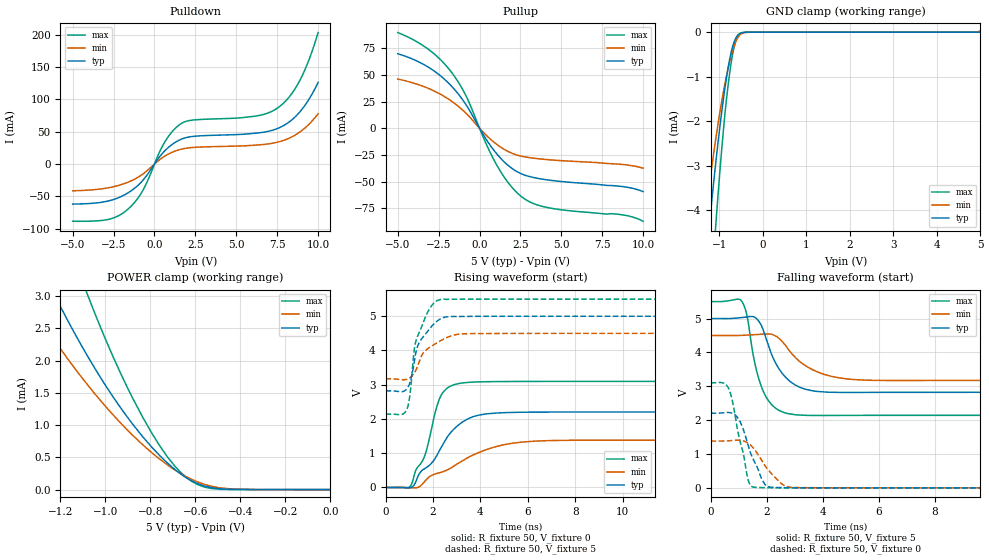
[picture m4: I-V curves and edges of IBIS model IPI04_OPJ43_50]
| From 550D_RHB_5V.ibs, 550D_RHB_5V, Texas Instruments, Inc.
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[Model]   IPI04_OPJ43_50
Model_type  I/O
Vinl = 0
Vinh = 5
Enable   Active-Low
Vref =   2.5
Rref =   50
Cref =   15p
Vmeas =   2.5
| variable   typ   min   max
C_comp   0.72pF   0.63pF   0.83pF
| C_pullup   1.77pF   0.56pF   2.42pF
| C_pulldown   1.53pF   0.86pF   2.26pF
| C_tri-state   0.72pF   0.63pF   0.83pF
[Temperature Range]   40   125   -40
| Ambient temperature   25   110   -40
[Voltage range]   5   4.5   5.5
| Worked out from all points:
|   slope of the pulldown table from 0 to 0.75 V, typ, clamps not added: 32.2 ohm
|   slope of the pullup table from 0 to 0.75 V, typ, clamps not added: 41.5 ohm
|   GND clamp passes 1 mA (typ) near -0.83 V on its own axis
|   POWER clamp passes 1 mA (typ) near -0.88 V on its own axis
|   rising waveform, R_fixture 50, V_fixture 0: 20-80 % time 1.51ns typ, 2.47ns min, 828ps max; typ from 0 V to 2.2 V
|   falling waveform, R_fixture 50, V_fixture 5: 20-80 % time 767ps typ, 1.13ns min, 547ps max; typ from 5 V to 2.82 V
|   rising waveform, R_fixture 50, V_fixture 5: 20-80 % time 679ps typ, 908ps min, 550ps max; typ from 2.82 V to 5 V
|   falling waveform, R_fixture 50, V_fixture 0: 20-80 % time 590ps typ, 746ps min, 451ps max; typ from 2.2 V to 0 V
[GND Clamp]
| IPI04_OPJ43_50
|   Voltage   I(typ)   I(min)   I(max)
-5V       -60.97mA   -47mA      -82.47mA
-1.345V   -5.553mA   -4.338mA   -8.207mA
-1.245V   -4.505mA   -3.561mA   -6.669mA
-1.205V   -4.104mA   -3.264mA   -6.077mA
-1.09V    -3.015mA   -2.458mA   -4.458mA
-1.055V   -2.704mA   -2.228mA   -3.994mA
-890mV    -1.395mA   -1.259mA   -2.04mA
-765mV    -627.7uA   -676.6uA   -948.2uA
-705mV    -363.7uA   -454uA     -561.7uA
-630mV    -151.5uA   -236uA     -226.2uA
-500mV    -18.16uA   -39.39uA   -19.17uA
5V        193pA      32.25uA    129.3pA
[POWER Clamp]
| IPI04_OPJ43_50
|   Voltage   I(typ)   I(min)   I(max)
-5V       60.35mA    45.31mA    80.38mA
-1.38V    4.15mA     3.131mA    6.161mA
-1.35V    3.917mA    2.964mA    5.812mA
-1.23V    3.04mA     2.33mA     4.491mA
-1.08V    2.071mA    1.626mA    3.023mA
-935mV    1.28mA     1.041mA    1.82mA
-835mV    822.7uA    697.6uA    1.127mA
-725mV    413.9uA    384.1uA    510.5uA
-635mV    172.1uA    190uA      174.4uA
-560mV    55.87uA    81.45uA    39.27uA
-490mV    12.95uA    27.01uA    5.254uA
-84.4fV   193pA      729pA      150.2pA
[Pulldown]
| IPI04_OPJ43_50
|   Voltage   I(typ)   I(min)   I(max)
-5V       -61.89mA   -41.4mA    -88.4mA
-2.815V   -57.01mA   -36.69mA   -85.54mA
-1.595V   -44.17mA   -27.83mA   -69.1mA
-685mV    -24.41mA   -14.96mA   -39.62mA
685mV     21.77mA    13.02mA    36.26mA
1.68V     38.72mA    23.14mA    63.14mA
6.295V    47.91mA    29.41mA    74.47mA
7.65V     56.24mA    34.57mA    88.8mA
8.3V      66.21mA    40.68mA    105.5mA
8.9V      80.88mA    49.68mA    129.8mA
9.46V     100.5mA    61.8mA     161.9mA
10V       126mA      77.5mA     203mA
[Pullup]
| IPI04_OPJ43_50
|   Voltage   I(typ)   I(min)   I(max)
-5V       69.87mA    46.14mA    89.69mA
-3.13V    57.25mA    37.38mA    74.02mA
-1.7V     39.22mA    25.25mA    52.2mA
-795mV    21.32mA    13.58mA    29.33mA
360mV     -9.264mA   -5.829mA   -13.14mA
1.06V     -24.13mA   -15.16mA   -34.71mA
1.825V    -35.8mA    -22.32mA   -52.46mA
2.6V      -42.96mA   -26.31mA   -64.49mA
3.275V    -46.05mA   -27.96mA   -70.42mA
4.195V    -48.49mA   -29.43mA   -74.43mA
8.695V    -54.54mA   -33.87mA   -81.04mA
10V       -59.36mA   -37.37mA   -87.19mA
[Ramp]
| IPI04_OPJ43_50
| variable   typ   min   max
dV/dt_r   1.33/1.52E-09   0.84/2.50E-09   1.86/8.41E-10
dV/dt_f   1.34/7.91E-10   0.82/1.16E-09   2.06/5.58E-10
R_load = 50
[Rising Waveform]
| IPI04_OPJ43_50
R_fixture =   50
C_fixture =   0
L_fixture =   0
V_fixture =   0
V_fixture_min = 0
V_fixture_max = 0
|   Time   V(typ)   V(min)   V(max)
0s        -402.9nV   -5.07uV    340.7nV
1.045ns   -5.03mV    -6.704mV   34.55mV
1.285ns   183.1mV    -8.556mV   515.3mV
1.68ns    565.1mV    201.2mV    981.7mV
2.075ns   832.2mV    390.3mV    2.144V
2.31ns    1.126V     437.9mV    2.644V
3.11ns    1.845V     724.3mV    3.038V
4.11ns    2.135V     1.069V     3.087V
6.405ns   2.201V     1.357V     3.097V
24.99ns   2.204V     1.382V     3.099V
[Falling Waveform]
| IPI04_OPJ43_50
R_fixture =   50
C_fixture =   0
L_fixture =   0
V_fixture =   5
V_fixture_min = 4.5
V_fixture_max = 5.5
|   Time   V(typ)   V(min)   V(max)
0s        5V         4.5V       5.5V
1.11ns    5.029V     4.502V     5.511V
1.3ns     5.048V     4.511V     5.076V
1.585ns   5.031V     4.524V     3.655V
1.89ns    4.632V     4.541V     2.831V
2.36ns    3.624V     4.464V     2.328V
2.925ns   3.088V     3.935V     2.17V
3.97ns    2.837V     3.374V     2.137V
5.505ns   2.819V     3.182V     2.141V
24.99ns   2.822V     3.173V     2.142V
[Rising Waveform]
| IPI04_OPJ43_50
R_fixture =   50
C_fixture =   0
L_fixture =   0
V_fixture =   5
V_fixture_min = 4.5
V_fixture_max = 5.5
|   Time   V(typ)   V(min)   V(max)
0s        2.822V     3.173V     2.142V
885ps     2.872V     3.158V     2.263V
1.025ns   3.058V     3.204V     2.688V
1.2ns     3.615V     3.333V     3.968V
1.3ns     4.011V     3.457V     4.322V
1.565ns   4.38V      3.902V     4.769V
1.865ns   4.638V     4.094V     5.228V
2.35ns    4.936V     4.296V     5.493V
3.675ns   4.997V     4.495V     5.499V
24.99ns   5V         4.5V       5.5V
[Falling Waveform]
| IPI04_OPJ43_50
R_fixture =   50
C_fixture =   0
L_fixture =   0
V_fixture =   0
V_fixture_min = 0
V_fixture_max = 0
|   Time   V(typ)   V(min)   V(max)
0s        2.204V     1.382V     3.101V
650ps     2.225V     1.39V      2.931V
790ps     2.201V     1.399V     2.514V
1.03ns    1.992V     1.409V     1.446V
1.33ns    1.285V     1.326V     266.6mV
1.53ns    829.7mV    1.171V     21.05mV
2ns       55.61mV    586.2mV    5.705mV
2.545ns   7.34mV     110.9mV    1.382mV
2.945ns   3.742mV    8.744mV    548.6uV
24.99ns   2.261uV    1.529uV    686.4nV
